| IBIS file 71v25761z_bg.ibs created by s2ibis2 version 1.1
| North Carolina State University Electronics Research Laboratory  1995
[IBIS ver]   2.1
[File name]   71v25761z_bg.ibs
[File Rev]   1.1
[Date]   8/16/00
[Source]   Integrated Device Technology, Inc.
[Notes]   1. Temperatures: typ=25C, min=70C, max=0C 2. Cemos10_3v
   process. 3. Ramp rates based on 50 ohm load.
[Copyright]   Copyright 2000, Integrated Device Technology, Inc. Integrated
   Device Technology, Inc. ("IDT") hereby grants the user of this
   IBIS model a non-exclusive, nontransferable license to use
   this IBIS model under the following terms. The user is granted
   this license only to use the IBIS model and is not granted
   rights to sell, copy (except as needed to run the IBIS model),
   rent, lease or sub-license the IBIS model in whole or in part,
   or in modified form to anyone. The User may modify the IBIS
   model to suit its specific applications, but rights to
   derivative works and such modifications shall belong to IDT.
   This IBIS model is provided on an AS IS" basis and IDT makes
   absolutely no warranty with respect to the information
   contained herein. IDT DISCLAIMS AND CUSTOMER WAIVES ALL
   WARRANTIES, EXPRESS AND IMPLIED, INCLUDING WARRANTIES OF
   MERCHANTABILITY AND FITNESS FOR A PARTICULAR PURPOSE. THE
   ENTIRE RISK AS TO QUALITY AND PERFORMANCE IS WITH THE USER
   ACCORDINGLY, IN NO EVENT SHALL IDT BE LIABLE FOR ANY DIRECT OR
   INDIRECT DAMAGES, WHETHER IN CONTRACT OR TORT, INCLUDING ANY
   LOST PROFITS OR OTHER INCIDENTAL, CONSEQUENTIAL, EXEMPLARY, OR
   PUNITIVE DAMAGES ARISING OUT OF THE USE OR APPLICATION OF THE
   IBIS model. Further, IDT reserves the right to make changes
   without notice to any product herein to improve reliability,
   function, or design. IDT does not convey any license under
   patent rights or any other intellectual property rights,
   including those of third parties. IDT is not obligated to
   provide maintenance or support for the licensed IBIS model.
|   Component idt71V25761Z
[Component]   idt71V25761Z
[Manufacturer]   Integrated Device Technology
|   This component uses the 119 BGA package (BG)
[Package]
| variable   typ   min   max
R_pkg   328m   103m   556m
L_pkg   5.4nH   2.8nH   20.4nH
C_pkg   2.1pF   1.06pF   4.4pF
[Pin]  signal_name   model_name   R_pin   L_pin   C_pin
A1   VDDQ   POWER
A2   A6   INPAD_71V25761Z
A3   A4   INPAD_71V25761Z
A4   NADSP   INPAD_71V25761Z
A5   A8   INPAD_71V25761Z
A6   A16   INPAD_71V25761Z
A7   VDDQ   POWER
B1   NC   NC
B2   CS0   INPAD_71V25761Z
B3   A3   INPAD_71V25761Z
B4   NADSC   INPAD_71V25761Z
B5   A9   INPAD_71V25761Z
B6   NCS1   INPAD_71V25761Z
B7   NC   NC
C1   NC   NC
C2   A7   INPAD_71V25761Z
C3   A2   INPAD_71V25761Z
C4   VDD   POWER
C5   A12   INPAD_71V25761Z
C6   A15   INPAD_71V25761Z
C7   NC   NC
D1   IO16   IOPAD25761Z
D2   IOP3   IOPAD25761Z
D3   VSS   GND
D4   NC   NC
D5   VSS   GND
D6   IOP2   IOPAD25761Z
D7   IO15   IOPAD25761Z
E1   IO17   IOPAD25761Z
E2   IO18   IOPAD25761Z
E3   VSS   GND
E4   NCE   INPAD_71V25761Z
E5   VSS   GND
E6   IO13   IOPAD25761Z
E7   IO14   IOPAD25761Z
F1   VDDQ   POWER
F2   IO19   IOPAD25761Z
F3   VSS   GND
F4   NOE   INPAD_71V25761Z
F5   VSS   GND
F6   IO12   IOPAD25761Z
F7   VDDQ   POWER
G1   IO20   IOPAD25761Z
G2   IO21   IOPAD25761Z
G3   NBW3   INPAD_71V25761Z
G4   NADV   INPAD_71V25761Z
G5   NBW2   INPAD_71V25761Z
G6   IO11   IOPAD25761Z
G7   IO10   IOPAD25761Z
H1   IO22   IOPAD25761Z
H2   IO23   IOPAD25761Z
H3   VSS   GND
H4   NGW   INPAD_71V25761Z
H5   VSS   GND
H6   IO9   IOPAD25761Z
H7   IO8   IOPAD25761Z
J1   VDDQ   POWER
J2   VDD   POWER
J3   NC   NC
J4   VDD   POWER
J5   NC   NC
J6   VDD   POWER
J7   VDDQ   POWER
K1   IO24   IOPAD25761Z
K2   IO26   IOPAD25761Z
K3   VSS   GND
K4   CLK   INCLK_71V25761Z
K5   VSS   GND
K6   IO6   IOPAD25761Z
K7   IO7   IOPAD25761Z
L1   IO25   IOPAD25761Z
L2   IO27   IOPAD25761Z
L3   NBW4   INPAD_71V25761Z
L4   NC   NC
L5   NBW1   INPAD_71V25761Z
L6   IO4   IOPAD25761Z
L7   IO5   IOPAD25761Z
M1   VDDQ   POWER
M2   IO28   IOPAD25761Z
M3   VSS   GND
M4   NBWE   INPAD_71V25761Z
M5   VSS   GND
M6   IO3   IOPAD25761Z
M7   VDDQ   POWER
N1   IO29   IOPAD25761Z
N2   IO30   IOPAD25761Z
N3   VSS   GND
N4   A1   INPAD_71V25761Z
N5   VSS   GND
N6   IO2   IOPAD25761Z
N7   IO1   IOPAD25761Z
P1   IO31   IOPAD25761Z
P2   IOP4   IOPAD25761Z
P3   VSS   GND
P4   A0   INPAD_71V25761Z
P5   VSS   GND
P6   IO0   IOPAD25761Z
P7   IOP1   IOPAD25761Z
R1   NC   NC
R2   A5   INPAD_71V25761Z
R3   NLBO   INPAD_71V25761Z
R4   VDD   POWER
R5   VDD   POWER
R6   A13   INPAD_71V25761Z
R7   NC   NC
T1   NC   NC
T2   NC   NC
T3   A10   INPAD_71V25761Z
T4   A11   INPAD_71V25761Z
T5   A14   INPAD_71V25761Z
T6   NC   NC
T7   ZZ   INPAD_71V25761Z
U1   VDDQ   POWER
U2   NC   NC
U3   NC   NC
U4   NC   NC
U5   NC   NC
U6   NC   NC
U7   VDDQ   POWER
U70   GNDQ   GND
| IOIN IOIN   dummy_model
| OC   OC   dummy_model
| IN   IN   dummy_model
| CLK  CLK   dummy_model
[Pin Mapping]  pulldown_ref   pullup_ref   gnd_clamp_ref   power_clamp_ref
A1   NC   EXTVDDQ
A2   EXTGNDQ   EXTVDDQ   EXTGND   EXTVDD
A3   EXTGNDQ   EXTVDDQ   EXTGND   EXTVDD
A4   EXTGNDQ   EXTVDDQ   EXTGND   EXTVDD
A5   EXTGNDQ   EXTVDDQ   EXTGND   EXTVDD
A6   EXTGNDQ   EXTVDDQ   EXTGND   EXTVDD
A7   NC   EXTVDDQ
B1   NC   NC   NC   NC
B2   EXTGNDQ   EXTVDDQ   EXTGND   EXTVDD
B3   EXTGNDQ   EXTVDDQ   EXTGND   EXTVDD
B4   EXTGNDQ   EXTVDDQ   EXTGND   EXTVDD
B5   EXTGNDQ   EXTVDDQ   EXTGND   EXTVDD
B6   EXTGNDQ   EXTVDDQ   EXTGND   EXTVDD
B7   NC   NC   NC   NC
C1   NC   NC   NC   NC
C2   EXTGNDQ   EXTVDDQ   EXTGND   EXTVDD
C3   EXTGNDQ   EXTVDDQ   EXTGND   EXTVDD
C4   NC   EXTVDD
C5   EXTGNDQ   EXTVDDQ   EXTGND   EXTVDD
C6   EXTGNDQ   EXTVDDQ   EXTGND   EXTVDD
C7   NC   NC   NC   NC
D1   EXTGNDQ   EXTVDDQ   EXTGND   EXTVDD
D2   EXTGNDQ   EXTVDDQ   EXTGND   EXTVDD
D3   EXTGND   NC
D4   NC   NC   NC   NC
D5   EXTGND   NC
D6   EXTGNDQ   EXTVDDQ   EXTGND   EXTVDD
D7   EXTGNDQ   EXTVDDQ   EXTGND   EXTVDD
E1   EXTGNDQ   EXTVDDQ   EXTGND   EXTVDD
E2   EXTGNDQ   EXTVDDQ   EXTGND   EXTVDD
E3   EXTGND   NC
E4   EXTGNDQ   EXTVDDQ   EXTGND   EXTVDD
E5   EXTGND   NC
E6   EXTGNDQ   EXTVDDQ   EXTGND   EXTVDD
E7   EXTGNDQ   EXTVDDQ   EXTGND   EXTVDD
F1   NC   EXTVDDQ
F2   EXTGNDQ   EXTVDDQ   EXTGND   EXTVDD
F3   EXTGND   NC
F4   EXTGNDQ   EXTVDDQ   EXTGND   EXTVDD
F5   EXTGND   NC
F6   EXTGNDQ   EXTVDDQ   EXTGND   EXTVDD
F7   NC   EXTVDDQ
G1   EXTGNDQ   EXTVDDQ   EXTGND   EXTVDD
G2   EXTGNDQ   EXTVDDQ   EXTGND   EXTVDD
G3   EXTGNDQ   EXTVDDQ   EXTGND   EXTVDD
G4   EXTGNDQ   EXTVDDQ   EXTGND   EXTVDD
G5   EXTGNDQ   EXTVDDQ   EXTGND   EXTVDD
G6   EXTGNDQ   EXTVDDQ   EXTGND   EXTVDD
G7   EXTGNDQ   EXTVDDQ   EXTGND   EXTVDD
H1   EXTGNDQ   EXTVDDQ   EXTGND   EXTVDD
H2   EXTGNDQ   EXTVDDQ   EXTGND   EXTVDD
H3   EXTGND   NC
H4   EXTGNDQ   EXTVDDQ   EXTGND   EXTVDD
H5   EXTGND   NC
H6   EXTGNDQ   EXTVDDQ   EXTGND   EXTVDD
H7   EXTGNDQ   EXTVDDQ   EXTGND   EXTVDD
J1   NC   EXTVDDQ
J2   NC   EXTVDD
J3   NC   NC   NC   NC
J4   NC   EXTVDD
J5   NC   NC   NC   NC
J6   NC   EXTVDD
J7   NC   EXTVDDQ
K1   EXTGNDQ   EXTVDDQ   EXTGND   EXTVDD
K2   EXTGNDQ   EXTVDDQ   EXTGND   EXTVDD
K3   EXTGND   NC
K4   EXTGNDQ   EXTVDDQ   EXTGND   EXTVDD
K5   EXTGND   NC
K6   EXTGNDQ   EXTVDDQ   EXTGND   EXTVDD
K7   EXTGNDQ   EXTVDDQ   EXTGND   EXTVDD
L1   EXTGNDQ   EXTVDDQ   EXTGND   EXTVDD
L2   EXTGNDQ   EXTVDDQ   EXTGND   EXTVDD
L3   EXTGNDQ   EXTVDDQ   EXTGND   EXTVDD
L4   NC   NC   NC   NC
L5   EXTGNDQ   EXTVDDQ   EXTGND   EXTVDD
L6   EXTGNDQ   EXTVDDQ   EXTGND   EXTVDD
L7   EXTGNDQ   EXTVDDQ   EXTGND   EXTVDD
M1   NC   EXTVDDQ
M2   EXTGNDQ   EXTVDDQ   EXTGND   EXTVDD
M3   EXTGND   NC
M4   EXTGNDQ   EXTVDDQ   EXTGND   EXTVDD
M5   EXTGND   NC
M6   EXTGNDQ   EXTVDDQ   EXTGND   EXTVDD
M7   NC   EXTVDDQ
N1   EXTGNDQ   EXTVDDQ   EXTGND   EXTVDD
N2   EXTGNDQ   EXTVDDQ   EXTGND   EXTVDD
N3   EXTGND   NC
N4   EXTGNDQ   EXTVDDQ   EXTGND   EXTVDD
N5   EXTGND   NC
N6   EXTGNDQ   EXTVDDQ   EXTGND   EXTVDD
N7   EXTGNDQ   EXTVDDQ   EXTGND   EXTVDD
P1   EXTGNDQ   EXTVDDQ   EXTGND   EXTVDD
P2   EXTGNDQ   EXTVDDQ   EXTGND   EXTVDD
P3   EXTGND   NC
P4   EXTGNDQ   EXTVDDQ   EXTGND   EXTVDD
P5   EXTGND   NC
P6   EXTGNDQ   EXTVDDQ   EXTGND   EXTVDD
P7   EXTGNDQ   EXTVDDQ   EXTGND   EXTVDD
R1   NC   NC   NC   NC
R2   EXTGNDQ   EXTVDDQ   EXTGND   EXTVDD
R3   EXTGNDQ   EXTVDDQ   EXTGND   EXTVDD
R4   NC   EXTVDD
R5   NC   EXTVDD
R6   EXTGNDQ   EXTVDDQ   EXTGND   EXTVDD
R7   NC   NC   NC   NC
T1   NC   NC   NC   NC
T2   NC   NC   NC   NC
T3   EXTGNDQ   EXTVDDQ   EXTGND   EXTVDD
T4   EXTGNDQ   EXTVDDQ   EXTGND   EXTVDD
T5   EXTGNDQ   EXTVDDQ   EXTGND   EXTVDD
T6   NC   NC   NC   NC
T7   EXTGNDQ   EXTVDDQ   EXTGND   EXTVDD
U1   NC   EXTVDDQ
U2   NC   NC   NC   NC
U3   NC   NC   NC   NC
U4   NC   NC   NC   NC
U5   NC   NC   NC   NC
U6   NC   NC   NC   NC
U7   NC   EXTVDDQ
U70   EXTGNDQ   NC
| Models and submodels in the file (3): IOPAD25761Z (I/O), INCLK_71V25761Z (Input), INPAD_71V25761Z (Input)
